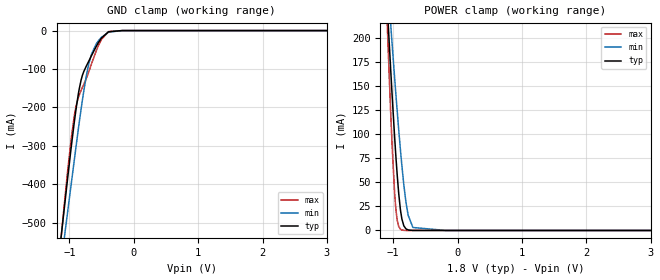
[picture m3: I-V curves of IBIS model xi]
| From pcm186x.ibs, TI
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|   xi Model
[Model]   xi
Model_type   Input
Vinl = 0.54
Vinh = 1.26
|   typ   min   max
|   (nom PVT)   (fast PVT)   (slow PVT)
C_comp   6.600e-12   6.533e-12   6.737e-12
[Model spec]
|subparameter
Vinl   0.54   0.486   0.594
Vinh   1.26   1.134   1.386
| Where nom  PVT is Nominal Process, 1.8V, 27C
|   Fast PVT is Strong Process,  1.98V, -40C
|   Slow PVT is Weak Process,   1.62V, 125C
[Voltage Range]   1.8   1.62   1.98
|Junction Temperature
[Temperature Range]   27   125   -40
[Power Clamp Reference]   1.8   1.62   1.98
[GND Clamp Reference]   0   0   0
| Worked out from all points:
|   GND clamp passes 1 mA (typ) near -0.25 V on its own axis
|   POWER clamp passes 1 mA (typ) near -0.78 V on its own axis
[GND Clamp]
|   Voltage   I(typ)   I(min)   I(max)
-1.8V     -1.603A    -1.519A    -1.756A
-1.186V   -624.4mA   -680.5mA   -635.3mA
-1.03V    -388.2mA   -475.5mA   -369.6mA
-968.9mV  -299.6mA   -396.1mA   -278mA
-891.2mV  -198.1mA   -294.8mA   -193mA
-819mV    -129.2mA   -205.2mA   -155.9mA
-698.4mV  -79.49mA   -86.54mA   -106.9mA
-657.9mV  -65.57mA   -61.76mA   -87.22mA
-580.3mV  -40.26mA   -33.9mA    -51.61mA
-502.4mV  -19.58mA   -17.61mA   -23.19mA
-393.8mV  -3.384mA   -4.346mA   -2.873mA
3.6V      0A         0A         0A
[POWER Clamp]
|   Voltage   I(typ)   I(min)   I(max)
-1.8V     1.221A     991.3mA    1.668A
-1.087V   228.3mA    261.1mA    206.6mA
-1.063V   198.3mA    238.5mA    164.7mA
-1.035V   163.9mA    212.1mA    118mA
-976.3mV  96.51mA    158.3mA    38.45mA
-936.7mV  57.54mA    124mA      10.68mA
-883.3mV  19.82mA    81.27mA    1.183mA
-834.5mV  4.929mA    47.78mA    127.1uA
-798.8mV  1.59mA     28.46mA    23.25uA
-766.4mV  541.9uA    15.81mA    4.925uA
-693.5mV  39.79uA    3.121mA    152.6nA
3.6V      0A         0A         0A
